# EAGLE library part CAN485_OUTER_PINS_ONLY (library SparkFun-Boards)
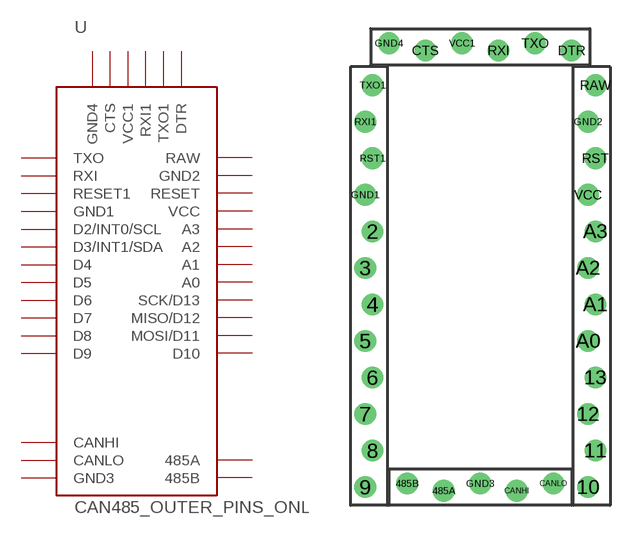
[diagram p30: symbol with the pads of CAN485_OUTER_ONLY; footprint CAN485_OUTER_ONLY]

Designator prefix -

## CAN485_OUTER_PINS_ONLY  [CAN485_OUTER_ONLY]
2  D2/INT0/SCL
3  D3/INT1/SDA
4  D4
5  D5
6  D6
7  D7
8  D8
9  D9
10  D10
11  MOSI/D11
12  MISO/D12
13  SCK/D13
485A  485A
485B  485B
A0  A0
A1  A1
A2  A2
A3  A3
CANHI  CANHI
CANLO  CANLO
CTS  CTS
DTR  DTR
GND1  GND1
GND2  GND2
GND3  GND3
GND4  GND4
RAW  RAW
RST  RESET
RST1  RESET1
RXI  RXI
RXI1  RXI1
TXO  TXO
TXO1  TXO1
VCC  VCC
VCC1  VCC1

## Footprint CAN485_OUTER_ONLY (pad centres in mm)
drill 1: 2 -7.493,0; 3 -8.001,-2.54; 4 -7.493,-5.08; 5 -8.001,-7.62; 6 -7.493,-10.16; 7 -8.001,-12.7; 8 -7.493,-15.24; 9 -8.001,-17.78; 10 7.493,-17.78; 11 8.001,-15.24; 12 7.493,-12.7; 13 8.001,-10.16; 485A -2.54,-18.034; 485B -5.08,-17.526; A0 7.493,-7.62; A1 8.001,-5.08; A2 7.493,-2.54; A3 8.001,0; CANHI 2.54,-18.034; CANLO 5.08,-17.526; CTS -3.81,12.573; DTR 6.35,12.573; GND1 -8.001,2.54; GND2 7.493,7.62; GND3 0,-17.526; GND4 -6.35,13.081; RAW 8.001,10.16; RST 8.001,5.08; RST1 -7.493,5.08; RXI 1.27,12.573; RXI1 -8.001,7.62; TXO 3.81,13.081; TXO1 -7.493,10.16; VCC 7.493,2.54; VCC1 -1.27,13.081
